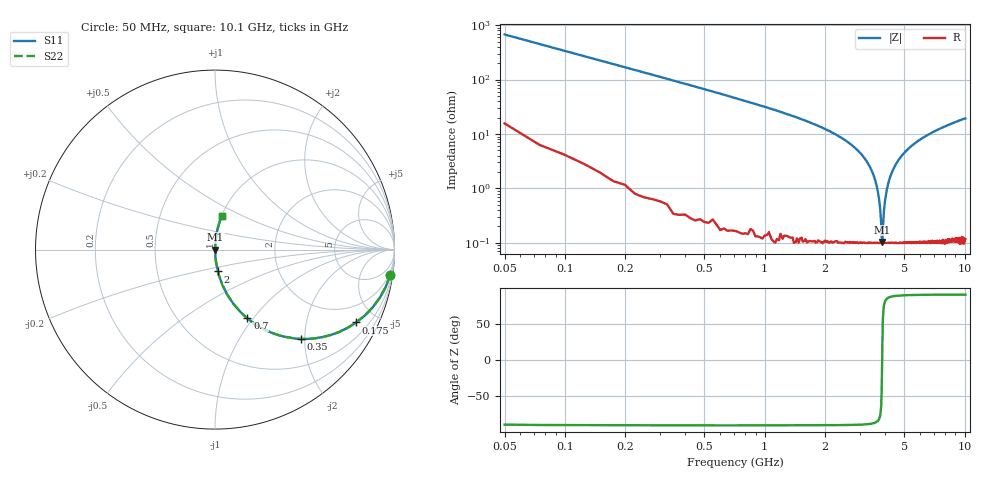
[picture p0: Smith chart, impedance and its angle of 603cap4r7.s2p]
! AVX Thin Film Operation		Date: November 2004
! Description: Accu-P® Series, Thin Film, SMD, RF Capacitor
! Part Number: 06035J4R7ABT
! 50 MHz  -  10.05 GHz
! Serial Measurements
# hz S db R 50
!	S11		S21		S12		S22
!	dB	Phase	dB	Phase	dB	Phase	dB	Phase
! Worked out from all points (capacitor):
!   400 points, 50 MHz to 10.1 GHz, reference 50 ohm
!   read as one part in series: C = 4.7 pF near 100 MHz
!   lowest |Z| = 103 mohm at 3.88 GHz (marker M1)
!   series resonance near 3.873 GHz, so ESL is about 360 pH
!   S11 on the Smith chart (normalised r, x): 50 MHz: 1, -14; 175 MHz: 1.03, -3.86; 350 MHz: 1.01, -1.92; 700 MHz: 1.00, -0.94; 2 GHz: 1.00, -0.25; 10.1 GHz: 1.00, +0.39
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5e7  -0.12 -8.4  -16.70 80.3  -16.70 80.3  -0.12 -8.4
1e8  -0.39 -16.4  -11.00 72.9  -11.00 72.9  -0.39 -16.4
1.75e8  -1.06 -27.3  -6.77 62.3  -6.77 62.3  -1.06 -27.3
3.5e8  -3.21 -46.1  -2.85 43.7  -2.85 43.7  -3.21 -46.1
7e8  -7.47 -64.8  -0.87 25.0  -0.87 25.0  -7.47 -64.8
1.73e9  -16.20 -80.7  -0.12 8.9  -0.12 8.9  -16.20 -80.7
2e9  -18.20 -82.4  -0.08 7.1  -0.08 7.1  -18.20 -82.4
2.93e9  -26.10 -86.0  -0.02 2.8  -0.02 2.8  -26.10 -86.0
3.4e9  -32.90 -86.2  -0.01 1.3  -0.01 1.3  -32.90 -86.2
3.73e9  -43.50 -81.1  -0.01 0.4  -0.01 0.4  -43.50 -81.1
3.78e9  -47.10 -76.7  -0.01 0.2  -0.01 0.2  -47.10 -76.7
3.83e9  -53.00 -63.4  -0.01 0.1  -0.01 0.1  -53.00 -63.4
3.85e9  -57.60 -41.0  -0.01 0.0  -0.01 0.0  -57.60 -41.0
3.88e9  -59.70 14.7  -0.01 -0.0  -0.01 -0.0  -59.70 14.7
3.95e9  -48.50 74.3  -0.01 -0.2  -0.01 -0.2  -48.50 74.3
4e9  -44.60 79.9  -0.01 -0.3  -0.01 -0.3  -44.60 79.9
4.2e9  -36.80 85.2  -0.01 -0.8  -0.01 -0.8  -36.80 85.2
4.6e9  -30.30 86.4  -0.01 -1.7  -0.01 -1.7  -30.30 86.4
5.08e9  -26.40 86.0  -0.02 -2.8  -0.02 -2.8  -26.40 86.0
6.75e9  -19.80 83.6  -0.05 -5.8  -0.05 -5.8  -19.80 83.6
8.43e9  -16.60 81.0  -0.11 -8.5  -0.11 -8.5  -16.60 81.0
1.01e10  -14.40 78.7  -0.17 -10.9  -0.17 -10.9  -14.40 78.7
